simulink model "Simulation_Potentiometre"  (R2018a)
settings: Solver=VariableStepAuto  StartTime=0.0  StopTime=340  RelTol=1e-3
libraries: simulink x1

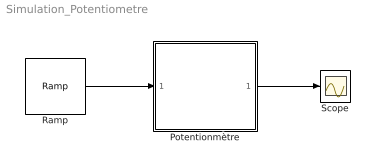
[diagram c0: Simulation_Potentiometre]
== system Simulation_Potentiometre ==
  Potentionmètre : Subsystem
  Ramp : simulink/Sources/Ramp  slope=1  start=0  InitialOutput=-170
  Scope : Scope
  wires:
  Ramp/1 -> Potentionmètre/1(Angle)
  Potentionmètre/1(Tension) -> Scope/1

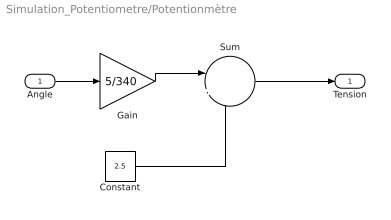
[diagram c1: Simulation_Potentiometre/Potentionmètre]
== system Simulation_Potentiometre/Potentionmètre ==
  Angle : Inport
  Constant : Constant  Value=2.5
  Gain : Gain  Gain=5/340
  Sum : Sum  Inputs=|++
  Tension : Outport
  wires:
  Constant/1 -> Sum/2
  Sum/1 -> Tension/1
  Angle/1 -> Gain/1
  Gain/1 -> Sum/1
